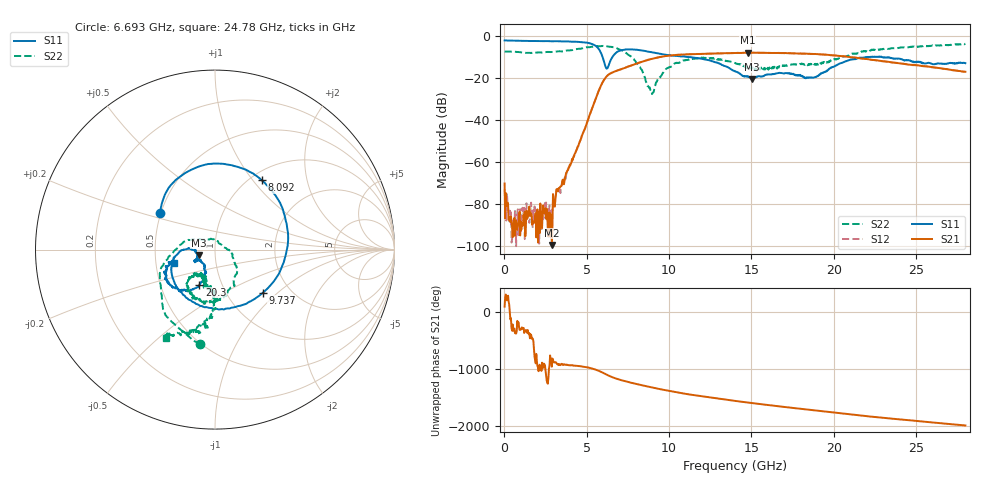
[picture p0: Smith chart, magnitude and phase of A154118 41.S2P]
!  2-Port S-parameters saved by WinCal
! VAR MeasName=S-Parameters (CALIBRATED_DATA) read from VNA (N5230A)
! VAR MeasDate=2015-9-10 14:37:37
! VAR NAME=A154118 41
! VAR FILENAME=A154118 41.S2P
! VAR DATE=2015-9-10 14:37:37
! VAR PHYS_PORTS=1,2
# Hz S DB R 50
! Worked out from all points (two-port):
!   801 points, 10 MHz to 28 GHz, reference 50 ohm
!   highest |S21| = -7.95 dB at 14.77 GHz (marker M1); lowest = -99.6 dB at 2.879 GHz (marker M2)
!   |S21| within 3 dB of the highest: 8.932 GHz to 21.96 GHz (13.03 GHz wide, 84.4 % of centre); 22.01426 GHz to 22.01819 GHz (3.928 MHz wide, 0.0178 % of centre)
!   lowest |S11| = -20.4 dB at 15.05 GHz (marker M3), VSWR 1.21, Z = 41.6 - j2.49 ohm
!   |S11| at or under -10 dB: 5.961 GHz to 6.557 GHz (595.8 MHz wide, 9.52 % of centre); 11.14 GHz to 22.04 GHz (10.9 GHz wide, 65.7 % of centre); 22.92 GHz to end of sweep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
!   |S22| runs from -27.7 to -3.7 dB; largest |S21 - S12| = 0.0071
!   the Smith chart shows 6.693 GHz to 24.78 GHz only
!   S11 on the Smith chart (normalised r, x): 6.693 GHz: 0.49, +0.24; 8.092 GHz: 1.13, +1.11; 9.737 GHz: 1.46, -0.81; 20.3 GHz: 0.78, -0.32; 24.78 GHz: 0.62, -0.10
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1e7  -2.15 179.7  -70.25 96.1  -72.92 130.8  -7.49 179.7
2.899e8  -2.19 175.7  -86.32 132.8  -88.22 -14.5  -7.45 171.1
2.878975e9  -2.53 140.3  -99.58 122.4  -82.87 69.3  -7.67 93.0
4.698325e9  -3.00 98.2  -47.59 126.3  -47.55 125.4  -5.94 13.3
5.293112e9  -3.76 69.7  -35.07 92.2  -35.08 92.0  -5.14 -18.7
5.74795e9  -6.43 26.6  -25.72 46.4  -25.72 46.3  -4.90 -43.4
6.1678e9  -15.11 -77.8  -19.60 -12.4  -19.58 -12.5  -4.83 -68.0
6.692612e9  -8.67 146.0  -16.93 -78.1  -16.95 -78.3  -5.44 -98.9
7.322388e9  -6.48 98.3  -15.18 -132.6  -15.18 -132.6  -7.62 -135.6
8.092112e9  -6.63 56.0  -12.95 172.8  -12.93 173.0  -13.69 176.9
8.931812e9  -7.74 7.0  -10.95 118.8  -10.93 118.9  -26.03 71.1
9.351662e9  -8.37 -19.1  -10.22 93.3  -10.16 93.2  -20.72 -9.6
9.736525e9  -8.91 -42.4  -9.63 71.1  -9.60 71.0  -16.34 -37.8
1.145091e10  -10.26 -125.8  -8.67 -15.8  -8.66 -16.5  -10.75 -89.5
1.4005e10  -16.76 176.6  -8.11 -118.9  -8.12 -119.3  -12.90 -131.7
1.477472e10  -19.43 -173.5  -7.95 -147.6  -7.91 -148.2  -14.96 -127.3
1.505462e10  -20.44 -161.8  -7.96 -157.6  -7.98 -158.2  -14.94 -124.8
1.869332e10  -19.79 -129.9  -8.54 78.2  -8.61 77.7  -13.08 -99.4
2.030275e10  -13.40 -114.0  -9.50 25.0  -9.46 23.9  -10.65 -91.1
2.334666e10  -10.31 -155.3  -12.33 -66.3  -12.34 -66.8  -6.18 -110.0
2.478115e10  -12.33 -161.7  -13.80 -103.8  -13.88 -104.8  -5.01 -119.0
2.8e10  -12.96 -154.3  -17.06 169.3  -17.14 168.5  -3.71 -138.1
